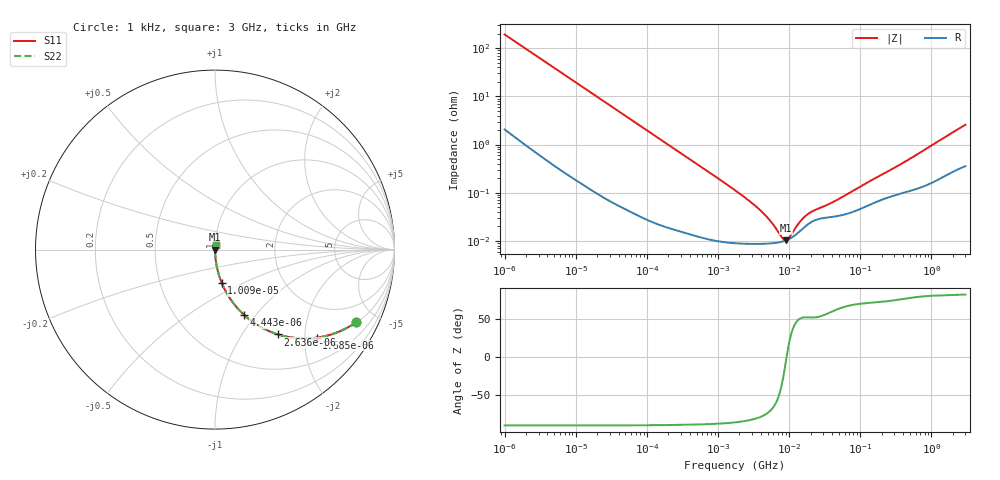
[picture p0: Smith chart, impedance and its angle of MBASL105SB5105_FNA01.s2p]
! MBASL105SB5105_FNA01  S-PARAMETER MODEL  ( Standard Model )
! Model Generated by TAIYO YUDEN Corporation (http://www.ty-top.com)
! Version 2.0
! TAIYO YUDEN Control No. 241120
! Copyright(c) 2013 TAIYO YUDEN CO.,LTD. All Rights Reserved.
! Product Description (link to TY-COMPAS)
! https://ds.yuden.co.jp/TYCOMPAS/or/detail?pn=MBASL105SB5105KFNA01&u=M
! Products Name : Multilayer Ceramic Capacitors
! Characteristics :
!  Capacitance : 1 [uF] , Rated Voltage : 10 [V] , TCC : X5R
!  Case Size : 1.0 x 0.5 / 0.039 x 0.02 [mm/inch] , Thickness : 0.5 / 0.02 [mm/inch]
!  (Conditions: Temperature = 25 [degC] , DC Bias Voltage = 0 [V])
! External Node Assignments :
!  1  o---| |---o  2
! GND o---------o GND
! Frequency Range : 1kHz  -  3GHz  [ 401 STEP ]
# MHZ S RI R 50
! Freq[MHz].  S11 Real  S11 Imag  S21 Real  S21 Imag  S12 Real  S12 Imag  S22 Real  S22 Imag
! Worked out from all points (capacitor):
!   401 points, 1 kHz to 3 GHz, reference 50 ohm
!   read as one part in series: C = 825 nF near 1.077 kHz
!   lowest |Z| = 10.3 mohm at 8.934 MHz (marker M1)
!   series resonance near 9.193 MHz, so ESL is about 360 pH
!   S11 on the Smith chart (normalised r, x): 1 kHz: 1.04, -3.85; 1.685 kHz: 1.02, -2.29; 2.636 kHz: 1.01, -1.47; 4.443 kHz: 1.01, -0.87; 10.09 kHz: 1.00, -0.39; 3 GHz: 1.01, +0.05
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0.001  0.7849 -0.4056  0.2151 0.4056  0.2151 0.4056  0.7849 -0.4056
0.001685  0.5671 -0.4905  0.4329 0.4905  0.4329 0.4905  0.5671 -0.4905
0.002636  0.3519 -0.4728  0.6481 0.4728  0.6481 0.4728  0.3519 -0.4728
0.004443  0.1628 -0.3645  0.8372 0.3645  0.8372 0.3645  0.1628 -0.3645
0.006451  0.0856 -0.2751  0.9144 0.2751  0.9144 0.2751  0.0856 -0.2751
0.010091  0.0377 -0.1857  0.9623 0.1857  0.9623 0.1857  0.0377 -0.1857
0.01216  0.0266 -0.1561  0.9734 0.1561  0.9734 0.1561  0.0266 -0.1561
0.033275  0.00408 -0.0587  0.9959 0.0587  0.9959 0.0587  0.00408 -0.0587
0.147855  0.000396 -0.0134  0.9996 0.0134  0.9996 0.0134  0.000396 -0.0134
1.732051  9.06e-05 -0.00112  0.9999 0.00112  0.9999 0.00112  9.06e-05 -0.00112
2.919173  8.7e-05 -0.000624  0.9999 0.000624  0.9999 0.000624  8.7e-05 -0.000624
4.238263  8.71e-05 -0.000378  0.9999 0.000378  0.9999 0.000378  8.71e-05 -0.000378
5.711239  8.92e-05 -0.000221  0.9999 0.000221  0.9999 0.000221  8.92e-05 -0.000221
7.988506  9.68e-05 -6.35e-05  0.9999 6.35e-05  0.9999 6.35e-05  9.68e-05 -6.35e-05
8.933959  0.000102 -1.29e-05  0.9999 1.29e-05  0.9999 1.29e-05  0.000102 -1.29e-05
9.991309  0.00011 3.77e-05  0.9999 -3.77e-05  0.9999 -3.77e-05  0.00011 3.77e-05
15.05716  0.000172 0.000217  0.9998 -0.000217  0.9998 -0.000217  0.000172 0.000217
17.47891  0.000209 0.00027  0.9998 -0.00027  0.9998 -0.00027  0.000209 0.00027
21.06097  0.000252 0.000322  0.9997 -0.000322  0.9997 -0.000322  0.000252 0.000322
44.39505  0.000322 0.000595  0.9997 -0.000595  0.9997 -0.000595  0.000322 0.000595
256.0921  0.00082 0.00276  0.9992 -0.00276  0.9992 -0.00276  0.00082 0.00276
3000  0.00418 0.0253  0.9958 -0.0253  0.9958 -0.0253  0.00418 0.0253
